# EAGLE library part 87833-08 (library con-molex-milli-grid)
HEADER
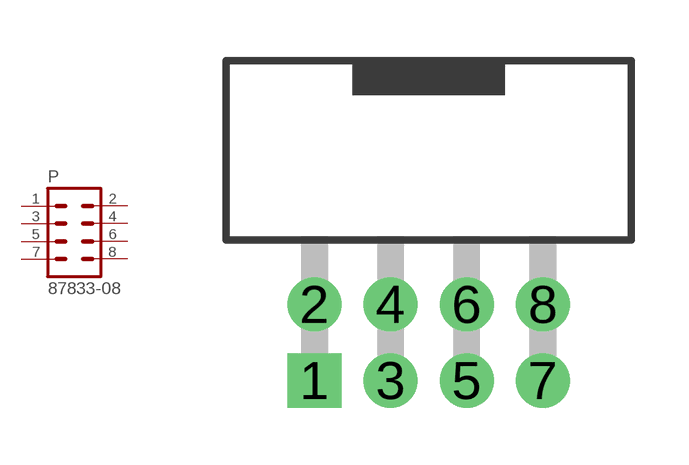
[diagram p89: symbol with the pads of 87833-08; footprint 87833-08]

Designator prefix P

## 87833-08  [87833-08]
1  1  pas
2  2  pas
3  3  pas
4  4  pas
5  5  pas
6  6  pas
7  7  pas
8  8  pas

## Footprint 87833-08 (pad centres in mm)
HEADER Dual Row, Shrouded, Right Angle
drill 0.914 square: 1 -3,-1
drill 0.914: 2 -3,1; 3 -1,-1; 4 -1,1; 5 1,-1; 6 1,1; 7 3,-1; 8 3,1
